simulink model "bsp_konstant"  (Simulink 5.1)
settings: Solver=ode45  SolverMode=SingleTasking  StartTime=0.0  StopTime=10.0  FixedStep=0.5  RelTol=1e-3
libraries: simulink x1

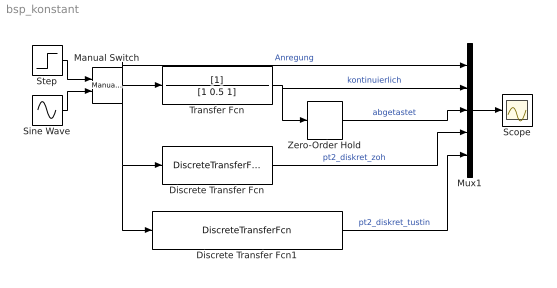
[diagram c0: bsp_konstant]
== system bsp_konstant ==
  Discrete Transfer Fcn : DiscreteTransferFcn  Numerator=[0.1129 0.1038]  Denominator=[1 -1.562 0.7788]  SampleTime=0.5
  Discrete Transfer Fcn1 : DiscreteTransferFcn  Numerator=[0.05263 0.1053 0.05263]  Denominator=[1 -1.579 0.7895]  SampleTime=0.5
  Manual Switch : simulink/Signal Routing/Manual Switch  sw=1  action=0
  Mux1 : Mux  Inputs=5
  Scope : Scope
  Sine Wave : Sin  SampleTime=0
  Step : Step  SampleTime=0
  Transfer Fcn : TransferFcn  Denominator=[1 0.5 1]
  Zero-Order Hold : ZeroOrderHold  SampleTime=0.5
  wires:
  Discrete Transfer Fcn/1 -> Mux1/4  "pt2_diskret_zoh"
  Mux1/1 -> Scope/1
  Transfer Fcn/1 -> Mux1/2, Zero-Order Hold/1  "kontinuierlich"
  Discrete Transfer Fcn1/1 -> Mux1/5  "pt2_diskret_tustin"
  Zero-Order Hold/1 -> Mux1/3  "abgetastet"
  Manual Switch/1 -> Transfer Fcn/1, Mux1/1, Discrete Transfer Fcn/1, Discrete Transfer Fcn1/1  "Anregung"
  Step/1 -> Manual Switch/1
  Sine Wave/1 -> Manual Switch/2
